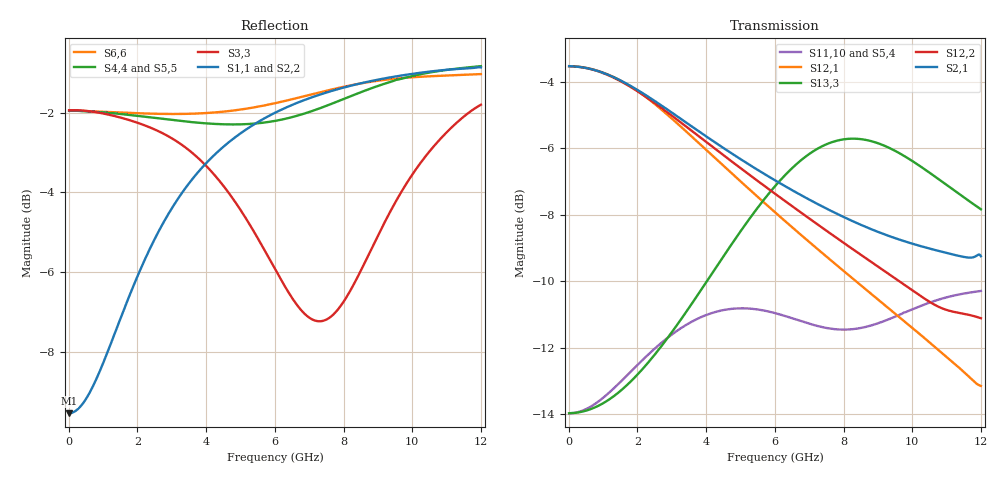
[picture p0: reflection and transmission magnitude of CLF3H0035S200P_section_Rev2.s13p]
! Touchstone file exported from HFSS 2020.2.0
!  File:  /home/rfpwrbs_nlv03685/HFSS/CLF3H0035S200P_Rev2/CLF3H0035S200P_section_Rev2.aedt
!  Generated:  2:40:43 PM  Jan 18, 2021
!  Design:  02_SOT467C1
!  Project:  CLF3H0035S200P_section_Rev2
!  Setup:  Setup1
!  Solution:  Sweep
! Variables:
!  AirBox_H = 20mm
!  AirBox_L = 30mm
!  AirBox_W = 60mm
!  pcb_h = 760um
# GHZ S MA R 50.000000
! Terminal data exported
! Port[1] = P9_BWT3_Rect_T1
! Port[2] = Box3_T1
! Port[3] = Box2_T1
! Port[4] = P1_BWT2_Rect_T1
! Port[5] = P2_BWT2_Rect_T1
! Port[6] = P3_BWT2_Rect_T1
! Port[7] = P4_BWT2_Rect_T1
! Port[8] = P5_BWT2_Rect_T1
! Port[9] = P6_BWT2_Rect_T1
! Port[10] = P7_BWT2_Rect_T1
! Port[11] = P8_BWT2_Rect_T1
! Port[12] = Rectangle2_T1
! Port[13] = Rectangle1_T1
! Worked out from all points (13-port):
!   1200 points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, 10 MHz to 12 GHz, reference 50 ohm
!   strongest paths, dB at 10 MHz, 3.01 GHz, 6.01 GHz, 9.01 GHz, 12 GHz:
!     S2,1: -3.5, -4.9, -7.0, -8.5, -9.2
!     S12,2: -3.5, -5.0, -7.4, -9.6, -11.1
!     S13,3: -14.0, -11.5, -7.1, -5.8, -7.8
!     S12,1: -3.5, -5.1, -7.9, -10.6, -13.2
!     S11,10: -14.0, -11.6, -11.0, -11.3, -10.3
!     S5,4: -14.0, -11.6, -11.0, -11.3, -10.3
!   lowest |S11| = -9.5 dB at 10 MHz (marker M1), VSWR 2.00, Z = 25 - j0.0728 ohm
!   |S11| at or under -10 dB: nowhere
